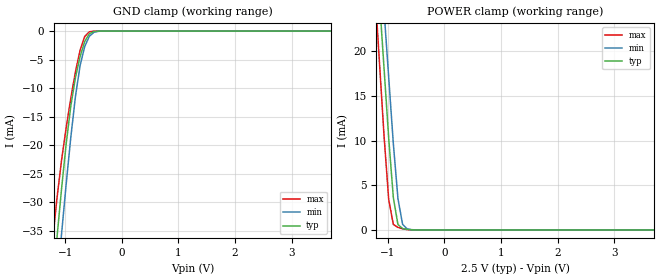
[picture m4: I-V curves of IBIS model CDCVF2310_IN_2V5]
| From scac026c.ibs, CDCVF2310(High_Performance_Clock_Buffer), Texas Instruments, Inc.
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[Model] CDCVF2310_IN_2V5
Model_type   Input
Polarity   Non-Inverting
Vinl = 0.800000   |--- Check this against the spec.
Vinh = 2.000000   |--- Check this against the spec.
| Variable   Typ   Min   Max
C_comp   2.0pF   NA   NA
|C_comp   2.0479e-12   2.0466e-12   2.0491e-12  |simulated Values
[Temperature range]   27   85   -40
[Voltage range]   2.5   2.3   2.7
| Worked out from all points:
|   GND clamp passes 1 mA (typ) near -0.60 V on its own axis
|   POWER clamp passes 1 mA (typ) near -0.83 V on its own axis
[GND Clamp]
|   Voltage   I(typ)   I(min)   I(max)
-2.7V     -222.5mA   -230.9mA   -213.5mA
-1.227V   -45.46mA   -54.06mA   -37.34mA
-1.145V   -36.37mA   -44.72mA   -29.42mA
-1.064V   -27.7mA    -35.61mA   -22.68mA
-981.8mV  -19.77mA   -26.84mA   -16.93mA
-900mV    -13.16mA   -18.64mA   -11.77mA
-818.2mV  -8.184mA   -11.48mA   -7.154mA
-736.4mV  -4.474mA   -6.071mA   -3.37mA
-654.5mV  -1.838mA   -2.709mA   -953.8uA
-572.7mV  -460.5uA   -910.4uA   -127.4uA
-327.3mV  -686.4nA   -5.007uA   -17.92nA
5.4V      14.97pA    672.5pA    32.13fA
[POWER Clamp]
|   Voltage   I(typ)   I(min)   I(max)
-2.7V     175.1mA    174.1mA    177.1mA
-1.227V   33.61mA    39.36mA    27.1mA
-1.145V   25.84mA    31.94mA    18.81mA
-1.064V   18.08mA    24.52mA    10.53mA
-981.8mV  10.31mA    17.1mA     3.441mA
-900mV    3.643mA    9.691mA    621.9uA
-818.2mV  607.3uA    3.513mA    289.3uA
-736.4mV  159.7uA    634.6uA    135.4uA
-654.5mV  63.04uA    115.2uA    42.45uA
-572.7mV  18.35uA    32.48uA    7.412uA
5.4V      -96.7pA    -4.104nA   -1.233pA
